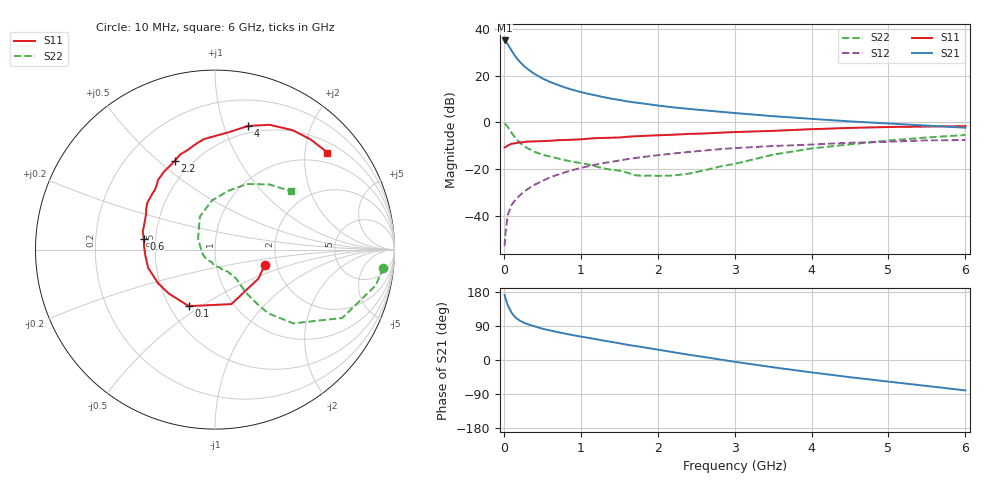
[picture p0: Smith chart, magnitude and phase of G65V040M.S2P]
! SIEMENS Small Signal Semiconductors
! BFG193
! Si NPN RF Bipolar Junction Transistor in SOT223
! VCE = 5 V  IC = 40 mA
! Common Emitter S-Parameters:  August  1996
# GHz  S  MA  R  50
!  f  S11  S21  S12  S22
! GHz  MAG  ANG  MAG  ANG  MAG  ANG  MAG  ANG
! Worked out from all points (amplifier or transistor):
!   36 points, 10 MHz to 6 GHz, reference 50 ohm
!   highest |S21| = 35.1 dB at 10 MHz (marker M1)
!   |S21| within 3 dB of that: start of sweep to 75.99 MHz
!   unconditionally stable (mu >= 1): 482.4 MHz to 2.426 GHz
!   at 250 MHz: K = 0.88, MSG = 27.3 dB, |S12| = -30.1 dB
!   at 1.4 GHz: K = 1.04, MAG = 12.3 dB, |S12| = -16.9 dB
!   at 6 GHz: K = 0.89, MSG = 2.7 dB, |S12| = -7.6 dB
!   S11 on the Smith chart (normalised r, x): 10 MHz: 1.73, -0.32; 100 MHz: 0.62, -0.45; 600 MHz: 0.43, +0.06; 2.2 GHz: 0.40, +0.57; 4 GHz: 0.43, +1.21; 6 GHz: 0.73, +2.50
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0.01  0.2903 -16.9  57.2 171.6  0.0022 88.2  0.9421 -6.1
0.02  0.2911 -33.6  55.25 164.6  0.004 87.3  0.918 -12.5
0.05  0.3172 -73.3  47.7 144.7  0.0102 72.8  0.8042 -28.3
0.1  0.3471 -114.9  34.82 124.9  0.017 65.5  0.5989 -43.3
0.15  0.3553 -136.5  25.93 112.1  0.0215 64.6  0.4611 -50.2
0.2  0.3687 -149.5  20.57 104.9  0.0264 66.7  0.3798 -52.2
0.25  0.375 -158.4  16.87 99.3  0.0312 66.2  0.3193 -53.6
0.3  0.3862 -164.7  14.29 95.0  0.036 67.5  0.2839 -54.3
0.4  0.3895 -175.1  10.91 88.7  0.0458 68.0  0.2326 -54.0
0.5  0.3959 177.5  8.778 82.7  0.0551 67.1  0.2023 -53.8
0.6  0.4013 171.3  7.375 78.1  0.0659 66.2  0.1845 -54.8
0.8  0.4178 161.1  5.556 69.4  0.0851 63.4  0.1533 -58.5
1.1  0.4458 149.3  4.084 58.4  0.1144 58.7  0.1241 -68.3
1.3  0.4627 141.5  3.469 51.1  0.1339 54.7  0.1025 -75.9
1.6  0.4899 131.1  2.821 40.4  0.1615 48.0  0.0836 -96.0
2.2  0.5426 114.5  2.099 20.7  0.2145 34.7  0.0721 -157.5
2.8  0.5987 100.1  1.695 1.7  0.2651 20.8  0.1118 147.9
3.5  0.6567 83.7  1.357 -19.2  0.3103 3.7  0.2027 114.5
4  0.7133 75.0  1.188 -32.7  0.3339 -6.1  0.2751 93.3
4.5  0.7587 66.4  1.049 -45.4  0.3646 -16.2  0.3372 76.9
5.5  0.8126 49.0  0.851 -68.5  0.4103 -39.5  0.4731 50.1
6  0.8278 40.8  0.767 -80.3  0.4163 -52.9  0.5346 37.3
